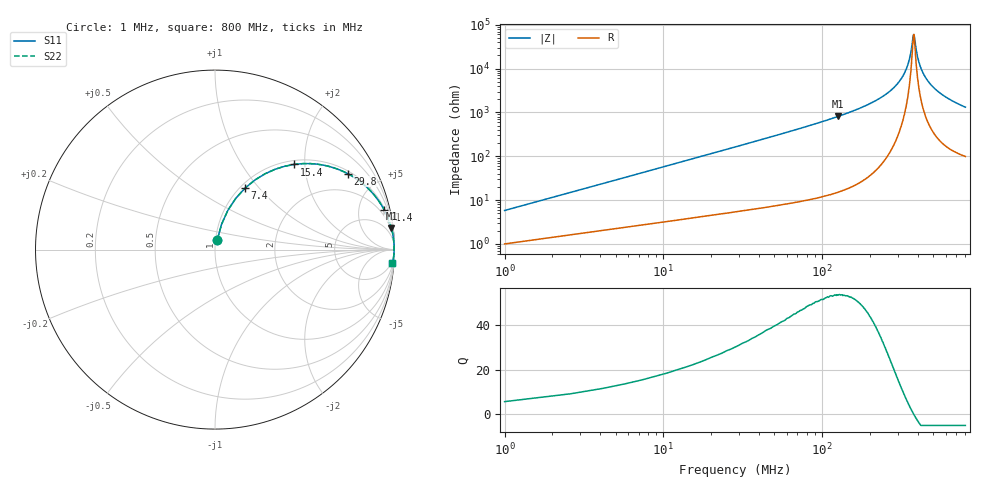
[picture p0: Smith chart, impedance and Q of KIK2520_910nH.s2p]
!version-2
!date-01.2022
!Series
# MHz S RI R 50
!Freq ReS11 ImS11 ReS21 ImS21 ReS12 ImS12 ReS22 ImS22
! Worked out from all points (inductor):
!   501 points, 1 MHz to 800 MHz, reference 50 ohm
!   read as one part in series: L = 910 nH near 4.2 MHz
!   highest Q = 53.7 at 126 MHz (marker M1), where L = 1.02 uH
!   self-resonance near 377 MHz
!   S11 on the Smith chart (normalised r, x): 1 MHz: 1.02, +0.11; 7.4 MHz: 1.05, +0.85; 15.4 MHz: 1.08, +1.76; 29.8 MHz: 1.11, +3.43; 71.4 MHz: 1.18, +8.47; 800 MHz: 3, -26
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1  0.0131 0.0559  0.9869 -0.0559  0.9869 -0.0559  0.0131 0.0559
5.8  0.1162 0.2862  0.8838 -0.2862  0.8838 -0.2862  0.1162 0.2862
7.4  0.1678 0.3429  0.8322 -0.3429  0.8322 -0.3429  0.1678 0.3429
15.4  0.4407 0.4746  0.5593 -0.4746  0.5593 -0.4746  0.4407 0.4746
29.8  0.7396 0.423  0.2604 -0.423  0.2604 -0.423  0.7396 0.423
45.8  0.8697 0.3238  0.1303 -0.3238  0.1303 -0.3238  0.8697 0.3238
71.4  0.9429 0.2215  0.0571 -0.2215  0.0571 -0.2215  0.9429 0.2215
126  0.9828 0.1212  0.0173 -0.1212  0.0173 -0.1212  0.9828 0.1212
135  0.9855 0.1107  0.0145 -0.1107  0.0145 -0.1107  0.9855 0.1107
268  0.9976 0.0323  0.00237 -0.0323  0.00237 -0.0323  0.9976 0.0323
307  0.9982 0.0195  0.00177 -0.0195  0.00177 -0.0195  0.9982 0.0195
339  0.9984 0.0103  0.00159 -0.0103  0.00159 -0.0103  0.9984 0.0103
358  0.9984 0.00516  0.00159 -0.00516  0.00159 -0.00516  0.9984 0.00516
377  0.9983 0.000347  0.00165 -0.000347  0.00165 -0.000347  0.9983 0.000347
382  0.9983 -0.000817  0.00168 0.000817  0.00168 0.000817  0.9983 -0.000817
391  0.9983 -0.0031  0.00174 0.0031  0.00174 0.0031  0.9983 -0.0031
401  0.9982 -0.00534  0.00181 0.00534  0.00181 0.00534  0.9982 -0.00534
423  0.998 -0.0103  0.00202 0.0103  0.00202 0.0103  0.998 -0.0103
447  0.9977 -0.0155  0.0023 0.0155  0.0023 0.0155  0.9977 -0.0155
534  0.9962 -0.0322  0.00376 0.0322  0.00376 0.0322  0.9962 -0.0322
667  0.993 -0.0544  0.00701 0.0544  0.00701 0.0544  0.993 -0.0544
800  0.9887 -0.0743  0.0112 0.0743  0.0112 0.0743  0.9887 -0.0743
